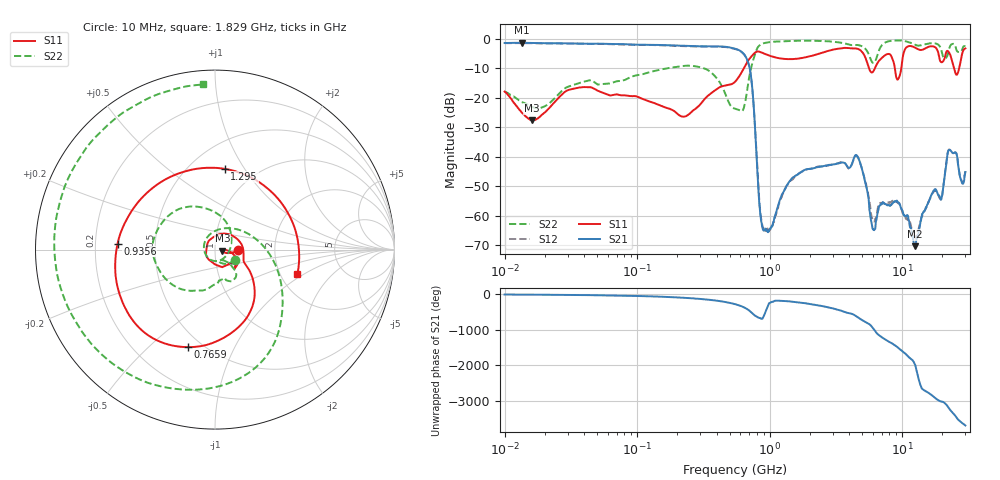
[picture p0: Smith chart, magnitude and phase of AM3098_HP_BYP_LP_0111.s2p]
!Agilent Technologies,E8364B,MY43040894,A.07.50.67
!Agilent E8364B: A.07.50.67
!Date: Wednesday, June 17, 2020 09:20:21
!Correction: S11(Full 2 Port(1,2))
!S21(Full 2 Port(1,2))
!S12(Full 2 Port(1,2))
!S22(Full 2 Port(1,2))
!S2P File: Measurements: S11, S21, S12, S22:Log Frequency Sweep
# Hz S  dB  R 50
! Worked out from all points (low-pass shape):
!   1601 points, 10 MHz to 30 GHz, reference 50 ohm
!   highest |S21| = -1.40 dB at 13.5 MHz (marker M1); lowest = -70.3 dB at 12.43 GHz (marker M2)
!   |S21| within 3 dB of the highest: start of sweep to 611.4 MHz
!   lowest |S11| = -27.6 dB at 16.01 MHz (marker M3), VSWR 1.09, Z = 54.3 - j0.592 ohm
!   |S11| at or under -10 dB: start of sweep to 639.8 MHz; 8.803 GHz to 9.852 GHz (1.048 GHz wide, 11.2 % of centre); 24.62 GHz to 26.93 GHz (2.306 GHz wide, 8.95 % of centre)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
!   |S22| runs from -24.6 to -0.6 dB; largest |S21 - S12| = 0.014
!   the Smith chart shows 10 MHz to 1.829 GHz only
!   S11 on the Smith chart (normalised r, x): 10 MHz: 1.29, -0.01; 765.9 MHz: 0.42, -0.67; 935.6 MHz: 0.30, +0.03; 1.295 GHz: 0.73, +0.82; 1.829 GHz: 2.48, -0.88
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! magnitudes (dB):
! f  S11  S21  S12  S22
! 10 MHz  -18.0  -1.5  -1.5  -18.0
! 13.5 MHz  -25.1  -1.4  -1.5  -21.5
! 16.01 MHz  -27.6  -1.5  -1.5  -23.1
! 38.04 MHz  -16.5  -1.7  -1.7  -14.8
! 144.7 MHz  -22.4  -2.1  -2.2  -10.6
! 333.7 MHz  -19.8  -2.6  -2.7  -10.4
! 547.7 MHz  -14.6  -3.4  -3.5  -23.7
! 689.5 MHz  -7.4  -8.1  -8.2  -14.9
! 765.9 MHz  -5.0  -25.9  -25.9  -6.1
! 850.8 MHz  -4.5  -59.6  -58.7  -2.1
! 935.6 MHz  -5.3  -64.4  -64.8  -1.4
! 1.295 GHz  -6.9  -51.2  -51.4  -0.8
! 1.829 GHz  -6.4  -44.6  -44.7  -0.7
! 2.084 GHz  -5.8  -44.0  -44.0  -0.7
! 4.525 GHz  -3.4  -39.5  -39.5  -2.1
! 6.019 GHz  -11.2  -64.5  -61.8  -8.2
! 7.926 GHz  -5.2  -56.3  -55.5  -0.9
! 9.302 GHz  -13.8  -55.4  -55.7  -0.7
! 12.43 GHz  -3.0  -70.3  -67.5  -2.0
! 19.7 GHz  -8.0  -54.5  -54.4  -3.7
! 22.67 GHz  -4.8  -37.7  -37.6  -3.3
! 30 GHz  -3.3  -45.2  -44.9  -2.6
